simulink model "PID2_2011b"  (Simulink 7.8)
settings: Solver=ode4  StartTime=0.0  StopTime=20  FixedStep=1e-2  RelTol=1e-3

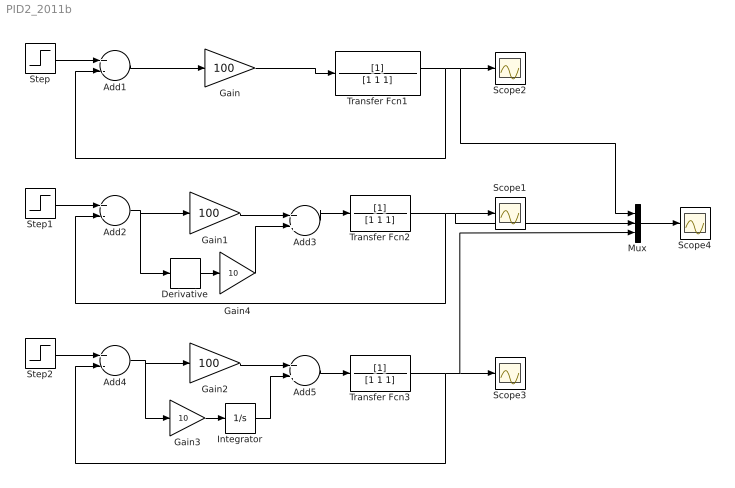
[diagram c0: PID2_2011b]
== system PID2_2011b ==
  Add1 : Sum  Inputs=+-
  Add2 : Sum  Inputs=+-
  Add3 : Sum
  Add4 : Sum  Inputs=+-
  Add5 : Sum
  Derivative : Derivative
  Gain : Gain  Gain=100
  Gain1 : Gain  Gain=100
  Gain2 : Gain  Gain=100
  Gain3 : Gain  Gain=10
  Gain4 : Gain  Gain=10
  Integrator : Integrator
  Mux : Mux  Inputs=3
  Scope{1..4} (4 alike) : Scope
  Step : Step  SampleTime=0
  Step1 : Step  SampleTime=0
  Step2 : Step  SampleTime=0
  Transfer Fcn1 : TransferFcn  Denominator=[1 1 1]
  Transfer Fcn2 : TransferFcn  Denominator=[1 1 1]
  Transfer Fcn3 : TransferFcn  Denominator=[1 1 1]
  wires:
  Step/1 -> Add1/1
  Transfer Fcn1/1 -> Add1/2, Scope2/1, Mux/1
  Add1/1 -> Gain/1
  Gain/1 -> Transfer Fcn1/1
  Step1/1 -> Add2/1
  Transfer Fcn2/1 -> Add2/2, Scope1/1, Mux/2
  Add2/1 -> Gain1/1, Derivative/1
  Add3/1 -> Transfer Fcn2/1
  Gain1/1 -> Add3/1
  Derivative/1 -> Gain4/1
  Step2/1 -> Add4/1
  Transfer Fcn3/1 -> Add4/2, Scope3/1, Mux/3
  Add4/1 -> Gain2/1, Gain3/1
  Add5/1 -> Transfer Fcn3/1
  Gain2/1 -> Add5/1
  Integrator/1 -> Add5/2
  Gain3/1 -> Integrator/1
  Mux/1 -> Scope4/1
  Gain4/1 -> Add3/2
